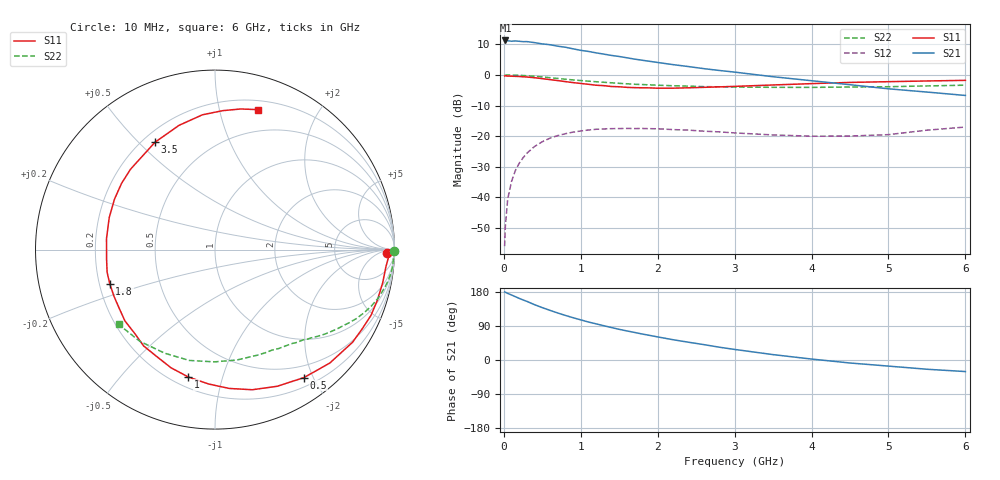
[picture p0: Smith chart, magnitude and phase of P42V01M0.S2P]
! SIEMENS Small Signal Semiconductors
! BFP182
! Si NPN RF Bipolar Junction Transistor in SOT143
! VCE = 2 V  IC = 1 mA
! Common Emitter S-Parameters:  March  1996
# GHz  S  MA  R  50
!  f  S11  S21  S12  S22
! GHz  MAG  ANG  MAG  ANG  MAG  ANG  MAG  ANG
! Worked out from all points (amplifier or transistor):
!   36 points, 10 MHz to 6 GHz, reference 50 ohm
!   highest |S21| = 11.3 dB at 20 MHz (marker M1)
!   |S21| within 3 dB of that: start of sweep to 953.7 MHz
!   unconditionally stable (mu >= 1): 2.593 GHz to end of sweep
!   at 250 MHz: K = 0.09, MSG = 19.0 dB, |S12| = -27.1 dB
!   at 1.4 GHz: K = 0.54, MSG = 12.0 dB, |S12| = -17.5 dB
!   at 6 GHz: K = 1.08, MAG = 3.4 dB, |S12| = -17.0 dB
!   S11 on the Smith chart (normalised r, x): 10 MHz: 41, -20; 500 MHz: 0.32, -1.87; 1 GHz: 0.26, -0.78; 1.8 GHz: 0.24, -0.15; 3.5 GHz: 0.25, +0.56; 6 GHz: 0.28, +1.31
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0.01  0.9611 -1.1  3.56 179.6  0.0016 88.7  0.9981 -0.4
0.02  0.968 -2.4  3.652 178.9  0.0034 88.4  0.9911 -0.8
0.05  0.9569 -5.8  3.61 175.8  0.0094 86.4  0.997 -2.1
0.1  0.9525 -11.1  3.55 171.5  0.0182 82.5  0.9942 -4.3
0.15  0.9476 -17.3  3.586 167.1  0.0275 79.3  0.9918 -6.5
0.3  0.924 -34.0  3.497 154.7  0.0527 68.7  0.9687 -12.6
0.4  0.8991 -44.7  3.364 145.9  0.068 62.7  0.9492 -16.4
0.5  0.8684 -55.2  3.209 138.2  0.0812 56.2  0.926 -19.9
0.6  0.8368 -65.5  3.111 131.0  0.0928 50.5  0.9017 -23.0
0.8  0.7775 -84.2  2.832 117.6  0.1097 40.2  0.8513 -28.6
1  0.7248 -101.9  2.518 105.9  0.1216 31.8  0.8097 -33.2
1.1  0.7027 -110.4  2.417 100.2  0.1261 28.0  0.7907 -35.3
1.3  0.6681 -126.5  2.184 90.4  0.1313 21.1  0.758 -39.1
1.5  0.6402 -141.6  1.999 80.9  0.1331 15.7  0.7284 -42.4
1.8  0.6165 -162.1  1.736 68.5  0.1335 9.1  0.696 -47.1
2.2  0.6076 174.2  1.472 53.5  0.128 2.3  0.6654 -53.7
2.8  0.6381 144.7  1.182 33.8  0.1175 -3.5  0.6394 -64.1
3.5  0.6852 119.2  0.934 14.2  0.1047 -3.3  0.627 -78.6
4  0.7209 106.1  0.804 2.5  0.0999 1.1  0.6256 -90.3
4.5  0.7544 95.3  0.692 -7.9  0.1004 5.6  0.634 -103.1
5.5  0.7966 79.6  0.525 -24.4  0.1253 15.0  0.6608 -129.4
6  0.8151 73.1  0.462 -30.5  0.1409 13.9  0.6798 -142.2
